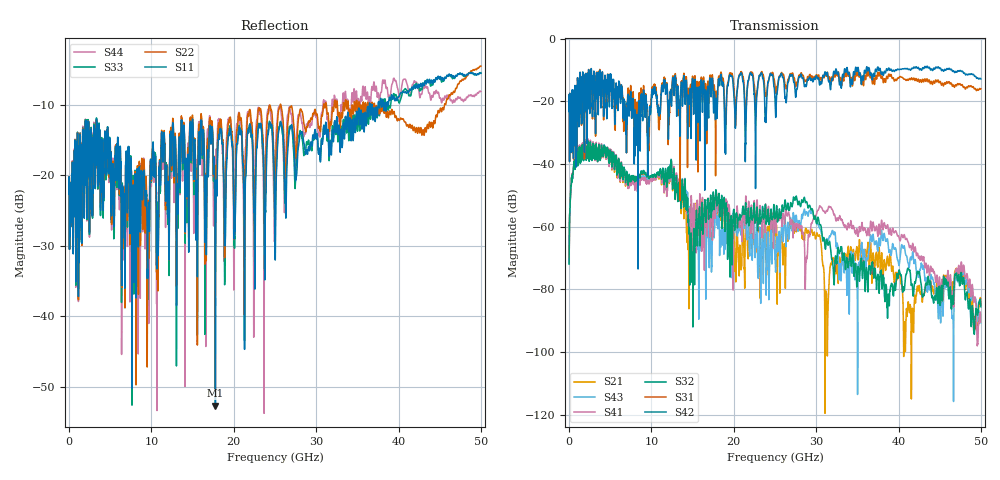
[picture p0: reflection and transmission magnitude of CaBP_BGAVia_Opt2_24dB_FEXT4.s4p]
!* Samtec Inc. NovaRay Examax Flyover System  *
!*  REV DATE  = 08/08/18  *
!*  TYPE  = TOUCHSTONE  *
!*  PORTS  = 4 port  *
!*  UNITS  = GHz  *
!*  DATA RANGE = DC  to 50 GHz; 10 MHz Step  *
!*  PARAMETER  = S  *
!*  FORMAT  = Real-Imaginary  *
!*  REFERENCE  = 50 ohms  *
!*  SOURCE  = HFSS  *
!*  VALIDATED  = No  *
!*  MANUFACTURER = SAMTEC  *
!*  INTERCONNECT = NVAx to EBCx to EBCx to NVAx  *
!*  [Full Channel NVAx to EBCx to EBCx to NVAx  with PCB Trace and BGA Via]  *
!*  BOUNDARY A  = Silicon BGA Ball Pad  *
!*  BOUNDARY B  = Silicon BGA Ball Pad  *
!*  NVAx (end a) ->>- (end b) NVAx  *
!*  Port 01 ->>- Port 02  *
!*  Port 03 ->>- Port 04  *
!***************************** CHANNEL MODEL ******************************************
# GHz S RI R 50
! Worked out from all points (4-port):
!   5000 points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, 10 MHz to 50 GHz, reference 50 ohm
!   strongest paths, dB at 10 MHz, 12.51 GHz, 25.01 GHz, 37.51 GHz, 50 GHz:
!     S42: -23.2, -14.8, -19.6, -9.1, -12.8
!     S31: -23.2, -14.5, -15.2, -10.7, -16.0
!     S32: -71.9, -44.0, -57.3, -75.5, -85.5
!     S41: -71.2, -43.0, -58.8, -62.7, -90.5
!     S43: -71.5, -43.0, -70.3, -67.0, -90.6
!     S21: -71.5, -44.0, -62.1, -71.8, -85.0
!   lowest |S11| = -52.7 dB at 17.77 GHz (marker M1), VSWR 1.00, Z = 49.8 - j0.145 ohm
!   |S11| at or under -10 dB: start of sweep to 36.46 GHz; 36.55 GHz to 36.75 GHz (204 MHz wide, 0.557 % of centre); 36.79 GHz to 37.51 GHz (722.9 MHz wide, 1.95 % of centre)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
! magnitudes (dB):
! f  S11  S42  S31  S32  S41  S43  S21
! 10 MHz  -22.7  -23.2  -23.2  -71.9  -71.2  -71.5  -71.5
! 2.1 GHz  -21.5  -19.6  -19.3  -38.2  -38.2  -38.3  -38.1
! 12.23 GHz  -18.1  -19.7  -22.9  -43.0  -43.7  -42.5  -43.9
! 14.87 GHz  -15.3  -19.4  -20.2  -69.6  -51.9  -54.2  -61.6
! 17.77 GHz  -52.7  -25.8  -28.1  -50.8  -55.9  -56.5  -54.1
! 31.27 GHz  -13.6  -11.2  -11.6  -64.1  -54.8  -63.8  -82.3
! 50 GHz  -5.5  -12.8  -16.0  -85.5  -90.5  -90.6  -85.0
